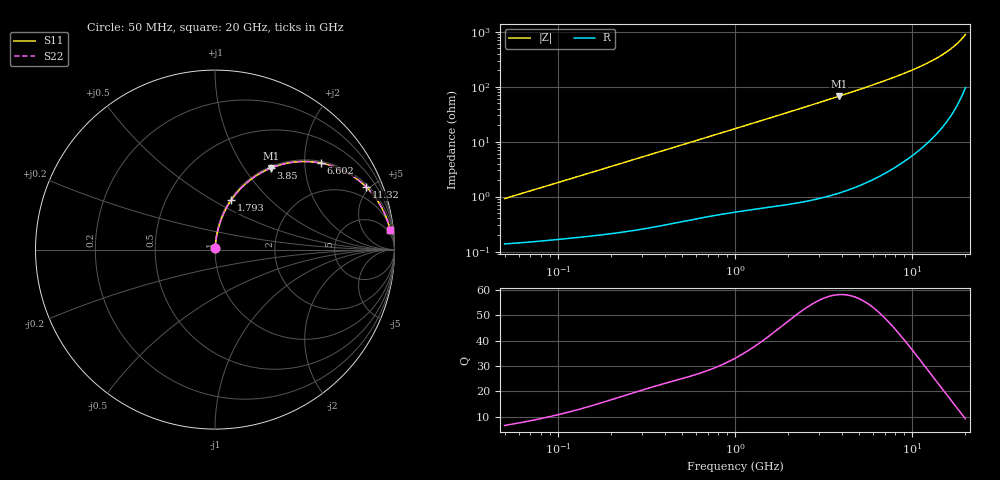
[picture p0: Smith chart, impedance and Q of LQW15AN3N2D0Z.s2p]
!Murata Part Number: LQW15AN3N2D0Z
!These Parameters are Measured in Series Mode Connection
!  o--[Z]--o
!Port1  Port2
!  o-------o
!Freq. Start=50[MHz] Stop=20[GHz], 401[Steps]
# Hz S RI R 50
!Freq.(Hz) S11(Real) S11(Imag) S21(Real) S21(Imag) S12(Real) S12(Imag) S22(Real) S22(Imag)
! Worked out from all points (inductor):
!   401 points, 50 MHz to 20 GHz, reference 50 ohm
!   read as one part in series: L = 2.88 nH near 51.52 MHz
!   highest Q = 58.1 at 3.85 GHz (marker M1), where L = 2.77 nH
!   S11 on the Smith chart (normalised r, x): 50 MHz: 1.00, +0.02; 1.793 GHz: 1.01, +0.61; 3.85 GHz: 1.02, +1.34; 6.602 GHz: 1.05, +2.40; 11.32 GHz: 1.15, +4.79; 20 GHz: 3, +18
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5e7  0.00146 0.00906  0.9985 -0.00906  0.9985 -0.00906  0.00146 0.00906
1.364002e8  0.00242 0.0242  0.9976 -0.0242  0.9976 -0.0242  0.00242 0.0242
3.721004e8  0.00707 0.0645  0.9929 -0.0645  0.9929 -0.0645  0.00707 0.0645
6.285508e8  0.0156 0.1068  0.9844 -0.1068  0.9844 -0.1068  0.0156 0.1068
1e9  0.0335 0.1653  0.9665 -0.1653  0.9665 -0.1653  0.0335 0.1653
1.369645e9  0.0573 0.2199  0.9427 -0.2199  0.9427 -0.2199  0.0573 0.2199
1.793498e9  0.0913 0.2772  0.9087 -0.2772  0.9087 -0.2772  0.0913 0.2772
2.211938e9  0.1307 0.3272  0.8693 -0.3272  0.8693 -0.3272  0.1307 0.3272
2.728004e9  0.1849 0.3791  0.8151 -0.3791  0.8151 -0.3791  0.1849 0.3791
3.216634e9  0.2396 0.4181  0.7604 -0.4181  0.7604 -0.4181  0.2396 0.4181
3.850025e9  0.3123 0.4549  0.6877 -0.4549  0.6877 -0.4549  0.3123 0.4549
5.117541e9  0.4513 0.4888  0.5487 -0.4888  0.5487 -0.4888  0.4513 0.4888
5.856089e9  0.5238 0.4902  0.4762 -0.4902  0.4762 -0.4902  0.5238 0.4902
6.601595e9  0.589 0.4822  0.411 -0.4822  0.411 -0.4822  0.589 0.4822
7.442007e9  0.6531 0.4655  0.3469 -0.4655  0.3469 -0.4655  0.6531 0.4655
9.316812e9  0.7637 0.4122  0.2363 -0.4122  0.2363 -0.4122  0.7637 0.4122
1.131968e10  0.844 0.3473  0.156 -0.3473  0.156 -0.3473  0.844 0.3473
1.354865e10  0.9024 0.277  0.0976 -0.277  0.0976 -0.277  0.9024 0.277
1.573793e10  0.9392 0.2136  0.0608 -0.2136  0.0608 -0.2136  0.9392 0.2136
1.774144e10  0.961 0.161  0.039 -0.161  0.039 -0.161  0.961 0.161
1.940974e10  0.973 0.1208  0.027 -0.1208  0.027 -0.1208  0.973 0.1208
2e10  0.9763 0.1074  0.0237 -0.1074  0.0237 -0.1074  0.9763 0.1074
